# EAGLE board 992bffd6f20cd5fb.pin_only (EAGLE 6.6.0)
REV: C

Size 50.8 x 22.86 mm. Coordinates in mm from the lower left corner, seen from the top.
Outline: 2.54,0 48.26,0 arc90 50.8,2.54 50.8,20.32 arc90 48.26,22.86 2.54,22.86 arc90 0,20.32 0,13.97 0.51,13.46 0.51,9.4 0,8.89 0,2.54 arc90 2.54,0
Copper layers (1*16): Top 0.035mm / dielectric 1.5mm / Bottom 0.035mm
Design rules "adafruit 7-7 *": minimum track width 6mil, minimum drill 15.5mil, track to track 8mil, track to pad 7mil, pad to pad 7mil, via to via 7mil, smd to smd 7mil, copper to edge 10mil, drill to drill 8mil, minimum pad ring 10mil, minimum via ring 8mil, stop-mask expansion 2mil, vias tented up to drill 20mil, thermal gap 10mil
Holes 2.2 mm at 48.26,1.84 48.26,20.95

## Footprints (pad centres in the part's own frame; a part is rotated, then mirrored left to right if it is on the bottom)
0805-NO = smd 1.24 x 1.5: 1 -0.95,0; 2 0.95,0
0603-NO = smd 1.075 x 1: 1 -0.85,0; 2 0.85,0
CHIPLED_0805_NOOUTLINE = smd 1.2 x 1.2: A 0,-1.05; C 0,1.05
SOD-123 = smd 1.4 x 1.4: A 1.85,0; C -1.85,0
QFN24_4MM_SMSC = smd 0.8 x 0.28: 1 -2,1.25; 2 -2,0.75; 3 -2,0.25; 4 -2,-0.25; 5 -2,-0.75; 6 -2,-1.25; 13 2,-1.25; 14 2,-0.75; 15 2,-0.25; 16 2,0.25; 17 2,0.75; 18 2,1.25 | smd 0.28 x 0.8: 7 -1.25,-2; 8 -0.75,-2; 9 -0.25,-2; 10 0.25,-2; 11 0.75,-2; 12 1.25,-2; 19 1.25,2; 20 0.75,2; 21 0.25,2; 22 -0.25,2; 23 -0.75,2; 24 -1.25,2 | smd 2.5 x 2.5: THERM 0,0
1X16_ROUND_MIN = drill 0.9 pad 1.575: 1 -19.05,0; 2 -16.51,0; 3 -13.97,0; 4 -11.43,0; 5 -8.89,0; 6 -6.35,0; 7 -3.81,0; 8 -1.27,0; 9 1.27,0; 10 3.81,0; 11 6.35,0; 12 8.89,0; 13 11.43,0; 14 13.97,0; 15 16.51,0; 16 19.05,0
1X12_ROUND_MIN = drill 0.9 pad 1.575: 1 -13.97,0; 2 -11.43,0; 3 -8.89,0; 4 -6.35,0; 5 -3.81,0; 6 -1.27,0; 7 1.27,0; 8 3.81,0; 9 6.35,0; 10 8.89,0; 11 11.43,0; 12 13.97,0
SOT23-3 = smd 0.8 x 0.9: 1 -0.95,-1; 2 0.95,-1; 3 0,1.1
SOT23-R = smd 0.635 x 1.016: 1 -0.95,-1; 2 0.95,-1; 3 0,1
RESPACK_4X0603 = smd 0.45 x 0.9: 1 -1.3,-0.85; 2 -0.4,-0.85; 3 0.4,-0.85; 4 1.3,-0.85; 5 1.3,0.85; 6 0.4,0.85; 7 -0.4,0.85; 8 -1.3,0.85
BTN_KMR2_4.6X2.8 = smd 0.9 x 0.9: A 2.05,0.8; A' -2.05,0.8; B 2.05,-0.8; B' -2.05,-0.8
SOT23-5 = smd 0.55 x 1.2: 1 -0.95,-1.3; 2 0,-1.3; 3 0.95,-1.3; 4 0.95,1.3; 5 -0.95,1.3
MOUNTINGHOLE_2.5_PLATED = drill 2.5 pad 3.2: P$1 0,0
FIDUCIAL_1MM = smd 1 x 1: 1 0,0
JSTPH2 = smd 1 x 4.6: 1 -1,-3.7; 2 1,-3.7 | smd 1.6 x 3.4: NC1 -3.4,1.5; NC2 3.4,1.5
WROOM32_SKINNY = smd 1.2 x 0.9: 1 -8.5,5; 2 -8.5,3.73; 3 -8.5,2.46; 4 -8.5,1.19; 5 -8.5,-0.08; 6 -8.5,-1.35; 7 -8.5,-2.62; 8 -8.5,-3.89; 9 -8.5,-5.16; 10 -8.5,-6.43; 11 -8.5,-7.7; 12 -8.5,-8.97; 13 -8.5,-10.24; 14 -8.5,-11.51; 25 8.5,-11.51; 26 8.5,-10.24; 27 8.5,-8.97; 28 8.5,-7.7; 29 8.5,-6.43; 30 8.5,-5.16; 31 8.5,-3.89; 32 8.5,-2.62; 33 8.5,-1.35; 34 8.5,-0.08; 35 8.5,1.19; 36 8.5,2.46; 37 8.5,3.73; 38 8.5,5 | smd 0.9 x 1.2: 15 -5.7,-12.9; 16 -4.43,-12.9; 17 -3.16,-12.9; 18 -1.89,-12.9; 19 -0.62,-12.9; 20 0.65,-12.9; 21 1.92,-12.9; 22 3.19,-12.9; 23 4.46,-12.9; 24 5.73,-12.9 | smd 6 x 6: P$1 0.34,-2.7
4UCONN_20329_V2 = smd 1 x 2: BASE@1 -0.75,-2; BASE@2 0.75,-2 | smd 0.4 x 1.35: D+ 0,0.775; D- -0.65,0.775; GND 1.3,0.775; ID 0.65,0.775; VBUS -1.3,0.775 | drill 0.8 pad 1.143 offset: SPRT@1 -3.3,0.9; SPRT@2 3.3,0.9 | drill 0.9 pad 2.413 square: SPRT@3 -3.6,-1.9; SPRT@4 3.6,-1.9 | hole 0.7: -1.95,0; 1.95,0

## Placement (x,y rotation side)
C1  10uF  [0805-NO]  11.68,4.9 270 top
C2  10uF  [0805-NO]  22.42,18.54 180 top
C3  10µF  [0805-NO]  16.13,18.03 270 top
C4  1uF  [0603-NO]  6.86,7.49 270 top
C6  10µF  [0805-NO]  18.92,18.88 180 top
C7  1uF  [0603-NO]  13.19,4.78 270 top
C8  10µF  [0805-NO]  14.37,12.89 270 top
CHG  ORANGE  [CHIPLED_0805_NOOUTLINE]  2.41,5.59 270 top
D3  RED  [CHIPLED_0805_NOOUTLINE]  2.86,17.34 90 top
D4  MBR120  [SOD-123]  9.78,12.19 180 top
IC1  CP2104  [QFN24_4MM_SMSC]  16.89,6.48 0 top
JP1  [1X16_ROUND_MIN]  25.4,1.27 180 top
JP3  [1X12_ROUND_MIN]  30.48,21.59 0 top
Q1  mmbt2222  [SOT23-3]  22.76,12.26 180 top
Q2  mmbt2222  [SOT23-3]  22.48,5.97 0 top
Q3  DMG3415U  [SOT23-R]  12.95,10.41 0 top
R1  100K  [0603-NO]  22.61,15.75 180 top
R2  1K  [0603-NO]  5.97,4.19 0 top
R3  100K  [0603-NO]  22.61,17.02 0 top
R4  4.7K  [0603-NO]  22.73,14.48 180 top
R7  100K  [0603-NO]  19.05,17.34 0 top
R10  1K  [0603-NO]  5.59,21.08 270 top
R12  100K  [0603-NO]  7.49,13.72 0 top
R13  10K  [RESPACK_4X0603]  22.54,9.14 0 top
SW2  KMR2  [BTN_KMR2_4.6X2.8]  9.14,6.22 270 top
U2  AP2112-3.3  [SOT23-5]  17.91,14.86 90 top
U3  MCP73831T-2ACI/OT  [SOT23-5]  17.91,11.56 270 top
U$7  [ADAFRUIT_5MM]  45.78,14.8 90 bottom
U$9  [FEATHERLOGO_MED]  24.13,7.49 0 bottom
U$13  [PCBFEAT-REV-040]  4.64,11.24 0 bottom
U$14  [ADAFRUIT_2.5MM]  11.73,6.45 0 top
U$15  [ADAFRUIT_3.5MM]  46.1,9.4 0 top
U$31  MOUNTINGHOLE2.5  [MOUNTINGHOLE_2.5_PLATED]  2.54,20.32 270 top
U$32  MOUNTINGHOLE2.5  [MOUNTINGHOLE_2.5_PLATED]  2.54,2.54 270 top
U$34  FIDUCIAL_1MM  [FIDUCIAL_1MM]  11.43,21.08 270 top
U$35  FIDUCIAL_1MM  [FIDUCIAL_1MM]  49.96,3.31 270 top
U$43  [HUZZAH32]  50.36,10.86 0 bottom
X1  JSTPH  [JSTPH2]  10.79,19.3 0 top
X2  ESP32_WROOM32_SKINNY  [WROOM32_SKINNY]  38.35,11.43 270 top
X4  20329  [4UCONN_20329_V2]  4.45,11.43 270 top

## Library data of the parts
C1-C4 C6 C7 CHG D3 D4 IC1 JP1 JP3 Q3 R1-R4 R7 R10 R12 R13 SW2 U2 U3 U$7 U$13-U$15 X1 X2 X4 = microbuilder
C8 = microbuilder; COMPANY: ADAFRUIT INDUSTRIES; DRAWN: KTOWN; REV: A
Q1 Q2 = SparkFun
U$9 U$43 = silks
U$31 U$32 U$34 U$35 = microbuilder; BOM: EXCLUDE

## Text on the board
tPlace: 12 | 27 | 33 | 15 | 32 | 14 | SCL | SDA | BAT | EN | USB | 13 | #13 | reset | huzzah! | CHG | ESP32! | RST | 3V | NC | GND | A0 | A1 | A2 | A3 | A4 | A5 | SCK | MO | MI | RX | TX | 21
bPlace: 3.7/4.2V / LiPoly Batt / µUSB charge | BAT | En | USB | 33/A9 | 15/A8 | 32/A7 | 14/A6 | 13/A12 | 12/A11 | 27/A10 | SCL/22 | SDA/23 | ESP32 Feather / 16MB Flash / WiFI+BT | Contains FCCID / 2AC7Z-ESP32 | MOSI/18 | MISO/19 | A1 / DAC1 | A2/34 | A3/39 | A4/36 | SCK/5 | RX/16 | TX/17 | RST | GND | A0 / DAC2 | A5/4 | 3V | NC | 21

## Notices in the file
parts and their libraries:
microbuilder: This work is placed in the public domain, and may be freely used for commercial and non-commercial work with the following conditions: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
SparkFun: Licensing: CC v3.0 Share-Alike You are welcome to use this library for commercial purposes.
